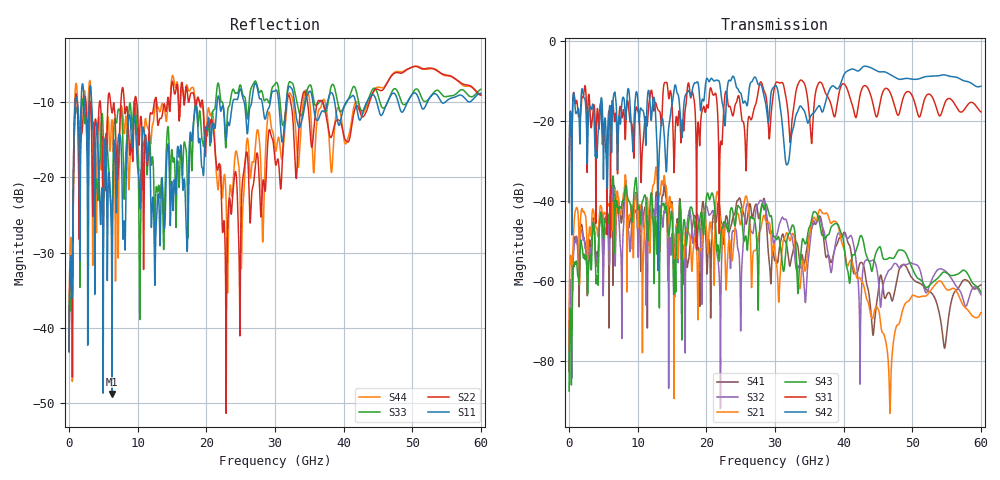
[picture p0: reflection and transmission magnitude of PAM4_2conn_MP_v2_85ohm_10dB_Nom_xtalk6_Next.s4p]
! Info: Touchstone file created by Circ.  Input file=FAB50GbE_2conn_Midplane_Examax_Topo2_v2_85ohm_10dB_Nom.circ
# Hz S RI R 50
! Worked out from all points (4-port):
!   6000 points, 10 MHz to 60 GHz, reference 50 ohm
!   strongest paths, dB at 10 MHz, 15.01 GHz, 30.01 GHz, 45.01 GHz, 60 GHz:
!     S42: -40.2, -15.9, -11.3, -7.7, -11.4
!     S31: -40.5, -16.3, -11.1, -18.2, -17.8
!     S43: -87.5, -43.9, -49.0, -52.0, -62.9
!     S21: -77.6, -41.0, -52.7, -67.0, -68.0
!     S32: -79.2, -48.4, -49.6, -59.0, -63.5
!     S41: -82.6, -40.7, -55.0, -63.1, -61.0
!   lowest |S11| = -48.8 dB at 6.26 GHz (marker M1), VSWR 1.01, Z = 50.3 + j0.166 ohm
!   |S11| at or under -10 dB: 3.284 GHz to 21.57 GHz (18.29 GHz wide, 147 % of centre); 21.93 GHz to 23.86 GHz (1.935 GHz wide, 8.45 % of centre); 35.52 GHz to 37.65 GHz (2.129 GHz wide, 5.82 % of centre)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
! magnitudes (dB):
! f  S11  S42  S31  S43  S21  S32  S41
! 10 MHz  -43.1  -40.2  -40.5  -87.5  -77.6  -79.2  -82.6
! 1.06 GHz  -9.4  -18.1  -15.0  -55.1  -41.8  -49.3  -48.9
! 6.26 GHz  -48.8  -21.6  -15.4  -36.3  -45.1  -39.7  -39.8
! 22.82 GHz  -14.9  -18.5  -12.7  -45.7  -59.4  -45.4  -44.2
! 36.65 GHz  -11.5  -16.9  -10.4  -47.1  -42.3  -44.9  -44.2
! 46.73 GHz  -9.4  -8.4  -12.8  -54.2  -92.0  -57.2  -63.2
! 60 GHz  -8.9  -11.4  -17.8  -62.9  -68.0  -63.5  -61.0
